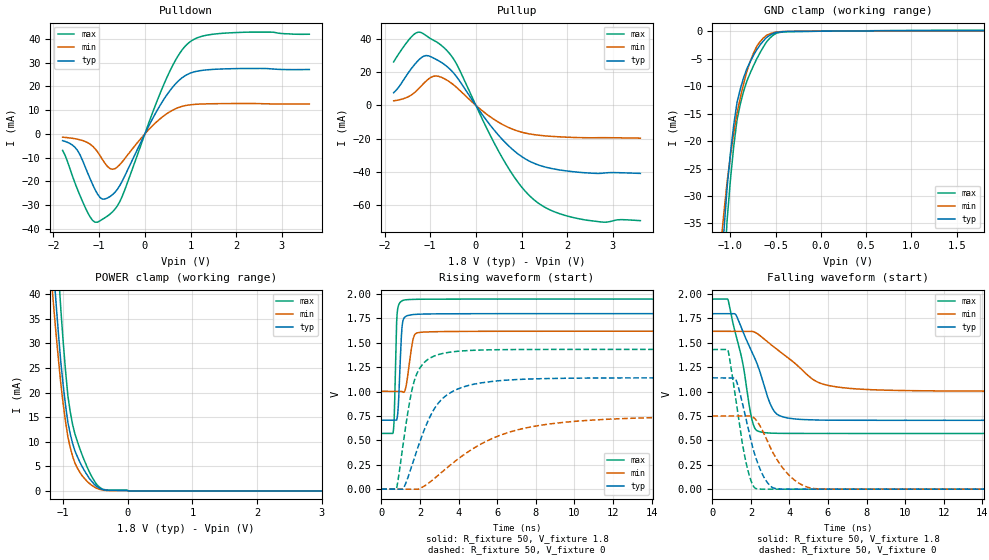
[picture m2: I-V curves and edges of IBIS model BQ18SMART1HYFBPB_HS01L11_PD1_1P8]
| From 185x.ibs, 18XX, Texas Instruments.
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|   Model Cell BQ18SMART1HYFBPB_HS01L11_PD1_1P8
|BQ18SMART1HYFBPB_HS01L11_PD1_1P8
[Model]   BQ18SMART1HYFBPB_HS01L11_PD1_1P8
Model_type   I/O
Polarity   Non-Inverting
Enable   Active-Low
Vinl =  0.63
Vinh =  1.17
Cref =  15pF
Rref =  100.0000M
Vref =  0V
Vmeas =  0.9
C_comp   0.915143p   0.8088923p   1.028577p
[Model Spec]
Vinl   0.63   0.567   0.6825
Vinh   1.17   1.053   1.2675
[Temperature Range]   25   125   -40
[Voltage Range]   1.8   1.62   1.95
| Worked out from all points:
|   slope of the pulldown table from 0 to 0.27 V, typ, clamps not added: 27.2 ohm
|   slope of the pullup table from 0 to 0.27 V, typ, clamps not added: 26 ohm
|   GND clamp passes 1 mA (typ) near -0.59 V on its own axis
|   POWER clamp passes 1 mA (typ) near -0.49 V on its own axis
|   rising waveform, R_fixture 50, V_fixture 1.8: 20-80 % time 144ps typ, 262ps min, 101ps max; typ from 0.707 V to 1.8 V
|   rising waveform, R_fixture 50, V_fixture 0: 20-80 % time 1.53ns typ, 3.82ns min, 759ps max; typ from 0 V to 1.14 V
|   falling waveform, R_fixture 50, V_fixture 1.8: 20-80 % time 1.25ns typ, 2.25ns min, 819ps max; typ from 1.8 V to 0.706 V
|   falling waveform, R_fixture 50, V_fixture 0: 20-80 % time 906ps typ, 1.34ns min, 687ps max; typ from 1.14 V to 0 V
| Nom Voltages:
|   BIASFET=1.8, VBBNW=1.1, VDD=1.1, VDDS=1.8, VSS=0, VSSS=0
| Min Voltages:
|   BIASFET=1.62, VBBNW=0.99, VDD=0.99, VDDS=1.62, VSS=0, VSSS=0
| Max Voltages:
|   BIASFET=1.95, VBBNW=1.21, VDD=1.21, VDDS=1.95, VSS=0, VSSS=0
[POWER_clamp]
|   voltage   I(typ)   I(min)   I(max)
-1.8V     196.9mA    157.5mA    250.4mA
-1.182V   51.67mA    43mA       68.61mA
-1.145V   44.45mA    37.16mA    60.1mA
-1.109V   37.9mA     31.74mA    52.07mA
-1.073V   31.79mA    26.6mA     44.33mA
-1.036V   26.12mA    21.74mA    36.87mA
-963.6mV  17.39mA    14.07mA    24.42mA
-927.3mV  13.91mA    10.96mA    19.29mA
-854.5mV  9.657mA    7.054mA    13.5mA
-709.1mV  4.995mA    3.131mA    7.393mA
-490.9mV  991uA      585.4uA    1.466mA
3.6V      0A         0A         0A
[Pulldown]
|   voltage   I(typ)   I(min)   I(max)
-1.8V     -2.835mA   -1.376mA   -6.938mA
-1.473V   -6.994mA   -2.229mA   -23.44mA
-1.2V     -18.79mA   -4.282mA   -34.89mA
-1.036V   -25.34mA   -7.531mA   -37.14mA
-872.7mV  -27.39mA   -12.36mA   -35.28mA
-654.5mV  -24.59mA   -14.63mA   -31.68mA
-490.9mV  -19.69mA   -11.65mA   -26.08mA
381.8mV   13.54mA    7.116mA    19.32mA
654.5mV   20.72mA    10.44mA    30.47mA
927.3mV   25mA       12.07mA    37.79mA
1.636V    27.3mA     12.74mA    42.26mA
3.6V      27.12mA    12.64mA    41.97mA
[Pullup]
|   voltage   I(typ)   I(min)   I(max)
-1.8V     7.614mA    2.74mA     26.22mA
-1.527V   17.69mA    4.626mA    37.43mA
-1.309V   25.69mA    8.541mA    43.72mA
-1.036V   29.87mA    15.94mA    41.05mA
-818.2mV  26.95mA    17.52mA    37.49mA
-490.9mV  19.61mA    12.45mA    28.08mA
545.5mV   -19.54mA   -10.94mA   -30.03mA
927.3mV   -29.38mA   -15.56mA   -46.58mA
1.255V    -34.7mA    -17.56mA   -56.51mA
1.691V    -38.25mA   -18.74mA   -63.85mA
2.291V    -40.42mA   -19.45mA   -68.55mA
3.6V      -41.01mA   -19.75mA   -69.5mA
[GND_clamp]
|   voltage   I(typ)   I(min)   I(max)
-1.8V     -274mA     -200.4mA   -365.5mA
-1.109V   -45.41mA   -39.33mA   -55.91mA
-1.073V   -36.49mA   -33.11mA   -44.46mA
-1.036V   -28.34mA   -27.37mA   -34.29mA
-1V       -22.19mA   -22.71mA   -27mA
-927.3mV  -12.97mA   -14.93mA   -16.12mA
-854.5mV  -8.452mA   -9.555mA   -10.93mA
-781.8mV  -5.549mA   -5.539mA   -7.634mA
-709.1mV  -3.363mA   -2.741mA   -5.028mA
-600mV    -1.121mA   -737.1uA   -1.924mA
-381.8mV  -62.21uA   -38.42uA   -93.33uA
1.8V      98.66uA    51.35uA    168.2uA
[Ramp]
| variable   typ   min   max
dV/dt_f 0.65734824/1.2499616n 0.37035125/2.2640357n 0.82843339/0.82184838n
dV/dt_r  0.6949594/1.5345628n 0.45752243/3.9311324n 0.86859566/0.76203805n
R_load = 50
[Rising Waveform]
R_fixture = 50
V_fixture = 1.8
V_fixture_min = 1.62
V_fixture_max = 1.95
|   time   V(typ)   V(min)   V(max)
0s        706.6mV    1.003V     571.3mV
614.6ps   706.6mV    1.003V     584.6mV
673.5ps   706.6mV    1.003V     770.5mV
767.6ps   706.6mV    1.003V     1.56V
815ps     722.4mV    1.003V     1.787V
1.113ns   1.719V     995.7mV    1.934V
1.282ns   1.772V     1.055V     1.941V
1.663ns   1.789V     1.549V     1.945V
1.913ns   1.793V     1.604V     1.946V
17.87ns   1.798V     1.619V     1.948V
[Rising Waveform]
R_fixture = 50
V_fixture = 0
V_fixture_min = 0
V_fixture_max = 0
|   time   V(typ)   V(min)   V(max)
0s        0V         0V         0V
779.1ps   0V         0V         0V
1.12ns    0V         0V         448.4mV
1.439ns   154.7mV    0V         864.2mV
1.686ns   304.1mV    0V         1.096V
2.064ns   524mV      13.72mV    1.261V
2.753ns   826.2mV    110mV      1.365V
4.291ns   1.05V      355.1mV    1.418V
7.543ns   1.128V     630mV      1.431V
18.05ns   1.141V     742.7mV    1.432V
[Falling Waveform]
R_fixture = 50
V_fixture = 1.8
V_fixture_min = 1.62
V_fixture_max = 1.95
|   time   V(typ)   V(min)   V(max)
0s        1.798V     1.618V     1.948V
817ps     1.798V     1.618V     1.938V
1.233ns   1.782V     1.618V     1.57V
1.598ns   1.608V     1.618V     1.271V
2.033ns   1.416V     1.618V     731.1mV
2.361ns   1.264V     1.59V      595.3mV
3.131ns   822.7mV    1.467V     573.5mV
3.925ns   729mV      1.347V     571.3mV
6.68ns    706.2mV    1.042V     571mV
17.87ns   705.8mV    1.004V     571mV
[Falling Waveform]
R_fixture = 50
V_fixture = 0
V_fixture_min = 0
V_fixture_max = 0
|   time   V(typ)   V(min)   V(max)
0s        1.14V      749.7mV    1.431V
811.1ps   1.14V      749.7mV    1.423V
1.222ns   1.12V      749.7mV    916.7mV
1.67ns    785mV      749.7mV    346.6mV
1.983ns   511mV      749.7mV    98.9mV
2.248ns   325.6mV    713.5mV    6.853mV
3.145ns   14.76mV    374.1mV    0V
4.088ns   0V         122.5mV    0V
5.095ns   0V         12.22mV    0V
18.05ns   0V         0V         0V
